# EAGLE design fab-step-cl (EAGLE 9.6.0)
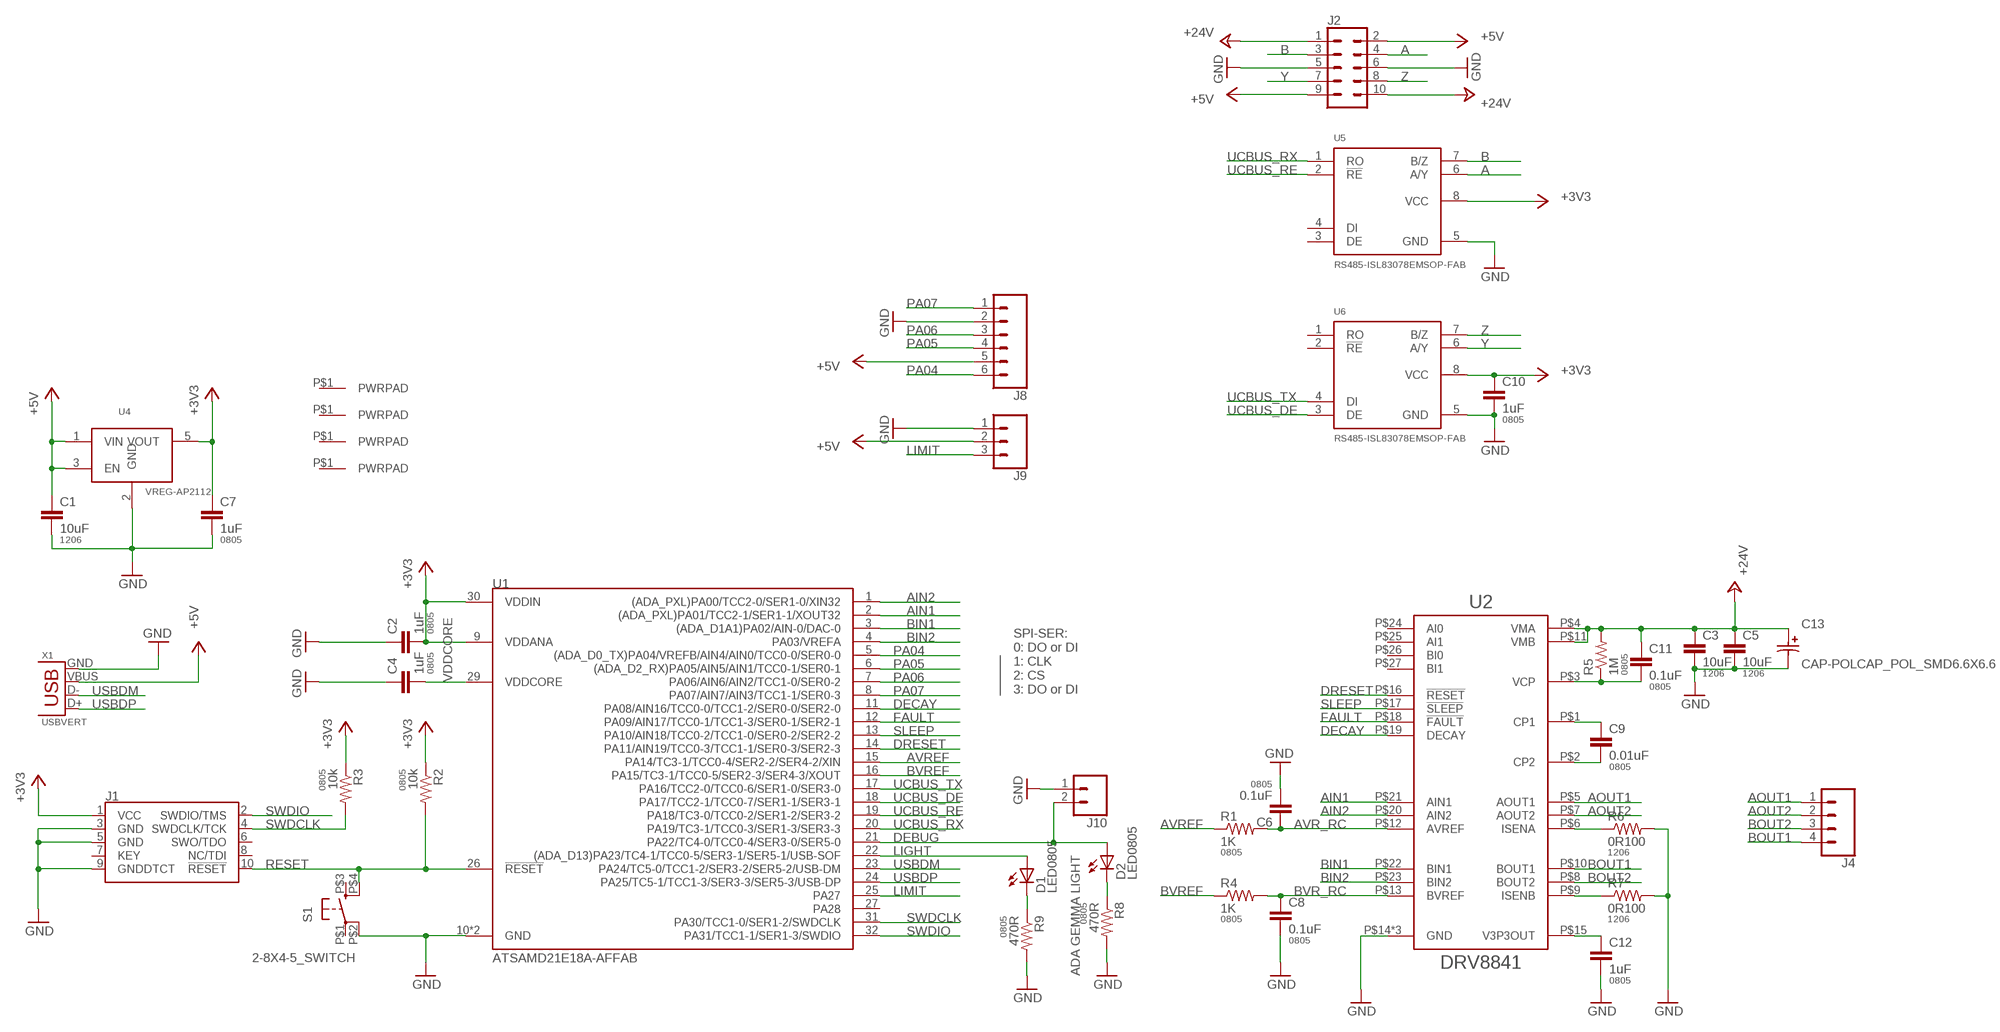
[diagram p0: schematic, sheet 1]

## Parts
C1  10uF  CAP1206  [1206]
C2  1uF  CAP0805  [0805]
C3  10uF  CAP1206  [1206]
C4  1uF  CAP0805  [0805]
C5  10uF  CAP1206  [1206]
C6  0.1uF  CAP0805  [0805]
C7  1uF  CAP0805  [0805]
C8  0.1uF  CAP0805  [0805]
C9  0.01uF  CAP0805  [0805]
C10  1uF  CAP0805  [0805]
C11  0.1uF  CAP0805  [0805]
C12  1uF  CAP0805  [0805]
C13  CAP-POLCAP_POL_SMD6.6X6.6  [SMD-ELEC-CAP]
D1  LED0805  [LED0805]
D2  LED0805  [LED0805]
J1  CORTEX_JTAG_DEBUG_PTH  [2X5-PTH-1.27MM]
J2  CONN_05X2SHD_LOCK_LATCH  [2X5-SHROUDED_LOCK_LATCH]
J3  PWRPADM3  [PWRPAD_3-25MM]
J4  CONN_041X04_NO_SILK  [1X04_NO_SILK]
J5  PWRPADM3  [PWRPAD_3-25MM]
J6  PWRPADM3  [PWRPAD_3-25MM]
J7  PWRPADM3  [PWRPAD_3-25MM]
J8  CONN_06NO_SILK_FEMALE_PTH  [1X06_NO_SILK]
J9  CONN_03JST-PTH-NS  [JST-3-PTH-NS]
J10  CONN_02LOCK  [1X02_LOCK]
R1  1K  RESISTOR0805-RES  [0805]
R2  10k  RESISTOR0805-RES  [0805]
R3  10k  RESISTOR0805-RES  [0805]
R4  1K  RESISTOR0805-RES  [0805]
R5  1M  RESISTOR0805-RES  [0805]
R6  0R100  RESISTOR1206  [1206]
R7  0R100  RESISTOR1206  [1206]
R8  470R  RESISTOR0805-RES  [0805]
R9  470R  RESISTOR0805-RES  [0805]
S1  2-8X4-5_SWITCH  [TACT-SWITCH-KMR6]
U1  ATSAMD21E18A-AFFAB  [TQFP-32-FAB]
U2  DRV8841  [HTSSOP-28]
U4  VREG-AP2112  [SOT23-5]
U5  RS485-ISL83078EMSOP-FAB  [8-MSOP-FAB]
U6  RS485-ISL83078EMSOP-FAB  [8-MSOP-FAB]
X1  USBVERT  [MOLEX_1051330021]

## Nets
+3V3: C2.2 C7.1 C10.1 J1.1(VCC) R2.1 R3.1 U1.9(VDDANA) U1.30(VDDIN) U4.5(VOUT) U5.8(VCC) U6.8(VCC)
+5V: C1.1 J2.2 J2.9 J8.5 J9.2 U4.1(VIN) U4.3(EN) X1.VBUS
+24V: C3.1 C5.1 C11.1 C13.A J2.1 J2.10 R5.2 U2.P$4(VMA) U2.P$11(VMB)
A: J2.4 U5.6(A/Y)
AIN1: U1.2((ADA_PXL)PA01/TCC2-1/SER1-1/XOUT32) U2.P$21(AIN1)
AIN2: U1.1((ADA_PXL)PA00/TCC2-0/SER1-0/XIN32) U2.P$20(AIN2)
AOUT1: J4.1 U2.P$5(AOUT1)
AOUT2: J4.2 U2.P$7(AOUT2)
AVR_RC: C6.1 R1.2 U2.P$12(AVREF)
AVREF: R1.1 U1.15(PA14/TC3-1/TCC0-4/SER2-2/SER4-2/XIN)
B: J2.3 U5.7(B/Z)
BIN1: U1.3((ADA_D1A1)PA02/AIN-0/DAC-0) U2.P$22(BIN1)
BIN2: U1.4(PA03/VREFA) U2.P$23(BIN2)
BOUT1: J4.4 U2.P$10(BOUT1)
BOUT2: J4.3 U2.P$8(BOUT2)
BVR_RC: C8.1 R4.2 U2.P$13(BVREF)
BVREF: R4.1 U1.16(PA15/TC3-1/TCC0-5/SER2-3/SER4-3/XOUT)
DEBUG: D2.1(A) J10.2 U1.21(PA22/TC4-0/TCC0-4/SER3-0/SER5-0)
DECAY: U1.11(PA08/AIN16/TCC0-0/TCC1-2/SER0-0/SER2-0) U2.P$19(DECAY)
DRESET: U1.14(PA11/AIN19/TCC0-3/TCC1-1/SER0-3/SER2-3) U2.P$16(!RESET)
FAULT: U1.12(PA09/AIN17/TCC0-1/TCC1-3/SER0-1/SER2-1) U2.P$18(!FAULT)
GND: C1.2 C2.1 C3.2 C4.1 C5.2 C6.2 C7.2 C8.2 C10.2 C12.2 C13.C J1.3(GND) J1.5(GND) J1.9(GNDDTCT) J2.5 J2.6 J8.2 J9.1 J10.1 R6.2 R7.2 R8.2 R9.2 S1.P$2(P1) U1.10(GND) U1.28(GND) U2.P$14(GND) U2.P$28(GND) U2.P$29(GND) U4.2(GND) U5.5(GND) U6.5(GND) X1.GND
ISENA: R6.1 U2.P$6(ISENA)
ISENB: R7.1 U2.P$9(ISENB)
LIGHT: D1.1(A) U1.22((ADA_D13)PA23/TC4-1/TCC0-5/SER3-1/SER5-1/USB-SOF)
LIMIT: J9.3 U1.25(PA27)
N$1: C9.2 U2.P$2(CP2)
N$2: C9.1 U2.P$1(CP1)
N$3: D2.2(C) R8.1
N$5: C11.2 R5.1 U2.P$3(VCP)
N$6: D1.2(C) R9.1
N$12: C12.1 U2.P$15(V3P3OUT)
PA04: J8.6 U1.5((ADA_D0_TX)PA04/VREFB/AIN4/AIN0/TCC0-0/SER0-0)
PA05: J8.4 U1.6((ADA_D2_RX)PA05/AIN5/AIN1/TCC0-1/SER0-1)
PA06: J8.3 U1.7(PA06/AIN6/AIN2/TCC1-0/SER0-2)
PA07: J8.1 U1.8(PA07/AIN7/AIN3/TCC1-1/SER0-3)
RESET: J1.10(!RESET) R2.2 S1.P$4(S1) U1.26(!RESET)
SLEEP: U1.13(PA10/AIN18/TCC0-2/TCC1-0/SER0-2/SER2-2) U2.P$17(!SLEEP)
SWDCLK: J1.4(SWDCLK/TCK) R3.2 U1.31(PA30/TCC1-0/SER1-2/SWDCLK)
SWDIO: J1.2(SWDIO/TMS) U1.32(PA31/TCC1-1/SER1-3/SWDIO)
UCBUS_DE: U1.18(PA17/TCC2-1/TCC0-7/SER1-1/SER3-1) U6.3(DE)
UCBUS_RE: U1.19(PA18/TC3-0/TCC0-2/SER1-2/SER3-2) U5.2(!RE)
UCBUS_RX: U1.20(PA19/TC3-1/TCC0-3/SER1-3/SER3-3) U5.1(RO)
UCBUS_TX: U1.17(PA16/TCC2-0/TCC0-6/SER1-0/SER3-0) U6.4(DI)
USBDM: U1.23(PA24/TC5-0/TCC1-2/SER3-2/SER5-2/USB-DM) X1.D-
USBDP: U1.24(PA25/TC5-1/TCC1-3/SER3-3/SER5-3/USB-DP) X1.D+
VDDCORE: C4.2 U1.29(VDDCORE)
Y: J2.7 U6.6(A/Y)
Z: J2.8 U6.7(B/Z)
Unconnected: J1.6(SWO/TDO) J1.7(KEY) J1.8(NC/TDI) J3.P$1(PWRPAD) J5.P$1(PWRPAD) J6.P$1(PWRPAD) J7.P$1(PWRPAD) S1.P$1(P) S1.P$3(S) U1.27(PA28) U2.P$24(AI0) U2.P$25(AI1) U2.P$26(BI0) U2.P$27(BI1) U5.3(DE) U5.4(DI) U6.1(RO) U6.2(!RE)

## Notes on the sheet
- SPI-SER:
  0: DO or DI
  1: CLK
  2: CS
  3: DO or DI
- ADA GEMMA LIGHT

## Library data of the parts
C1 C3 C5 = passives:CAP: Capacitor; PACKAGE: 1206
C2 C4 C6-C12 = passives:CAP: Capacitor; PACKAGE: 0805
C13 = passives:CAP-POL
D1 D2 = lights:LED: LED
J1 = SparkFun-Connectors:CORTEX_JTAG_DEBUG: Cortex Debug Connector - 10 pin Supports JTAG debug, Serial Wire debug, and Serial Wire Viewer. PTH and SMD connector options available. General Connector Information Products: PTH Connector -via Digi-Key SparkFun PSoc SparkFun T
J2 = SparkFun-Connectors:CONN_05X2: Multi connection point. Often used as Generic Header-pin footprint for 0.1 inch spaced/style header connections For AVR SPI programming port, see special device with nice symbol: "AVR_SPI_PROG_5x2.dev" You can populate with any combo of single row headers, but if you'd like an exact match, check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
J3 J5-J7 = connector:PWRPAD
J4 = SparkFun-Connectors:CONN_04: Multi connection point. Often used as Generic Header-pin footprint for 0.1 inch spaced/style header connections On any of the 0.1 inch spaced packages, you can populate with these: Break Away Headers - Straight (PRT-00116) Break Away Male Headers - Right Angle (PRT-00553) Female Headers (PRT-00115)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; PROD_ID: CONN-09696
J8 = SparkFun-Connectors:CONN_06: Multi connection point. Often used as Generic Header-pin footprint for 0.1 inch spaced/style header connections On any of the 0.1 inch spaced packages, you can populate with these: Break Away Headers - Straight (PRT-00116) Break Away Male Headers - Right Angle (PRT-00553) Female Headers (PRT-00115)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; PROD_ID: CONN-08437
J9 = SparkFun-Connectors:CONN_03: Multi connection point. Often used as Generic Header-pin footprint for 0.1 inch spaced/style header connections On any of the 0.1 inch spaced packages, you can populate with these: Break Away Headers - Straight (PRT-00116) Break Away Male Headers - Right Angle (PRT-00553) Female Headers (PRT-00115)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
J10 = SparkFun-Connectors:CONN_02: Multi connection point. Often used as Generic Header-pin footprint for 0.1 inch spaced/style header connections
R1-R5 R8 R9 = passives:RESISTOR: Resistor; PACKAGE: 0805
R6 R7 = passives:RESISTOR: Resistor; PACKAGE: 1206
S1 = passives:2-8X4-5_SWITCH
U1 = microcontrollers:ATSAMD21E18A-AF: The SAM D21 is a series of low-power microcontrollers using the 32-bit ARM® Cortex® -M0+ processor, and ranging from 32- to 64-pins with up to 256KB Flash and 32KB of SRAM. The SAM D21 operate at a maximum frequency of 48MHz and reach 2.46 CoreMark® /MHz. Check prices
U2 = power:DRV8841
U4 = power:VREG-AP2112
U5 U6 = comm:RS485-ISL83078E
X1 = connector:USB: SMD micro USB connector as found in the fablab inventory. Three footprint variants included: 609-4613-1-ND used by Jake original, as described by manufacturer's datasheet for milling with the 1/100" bit for milling with the 1/64" bit Made by Zaerc.

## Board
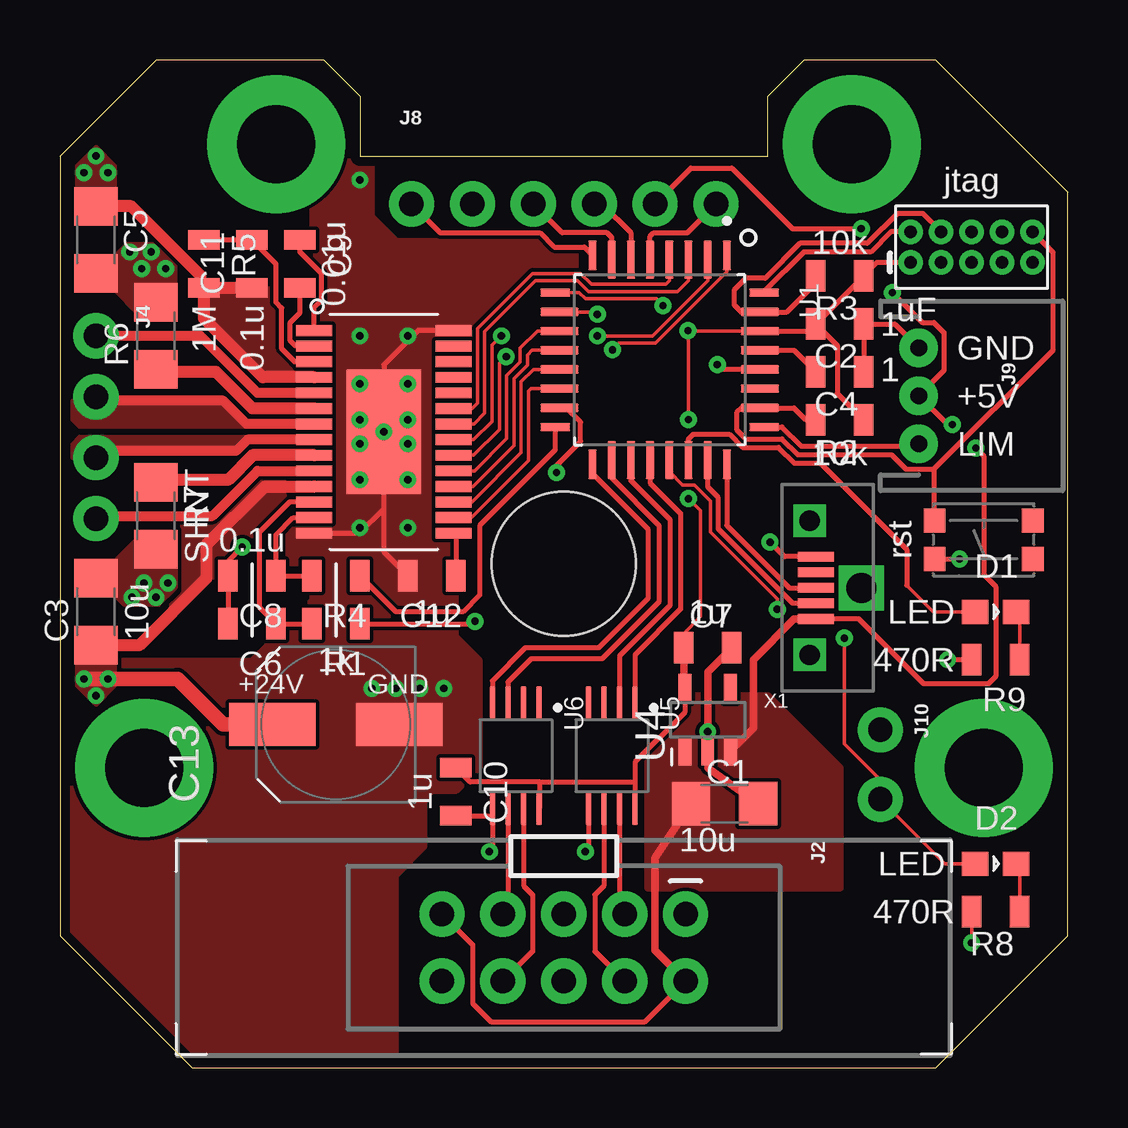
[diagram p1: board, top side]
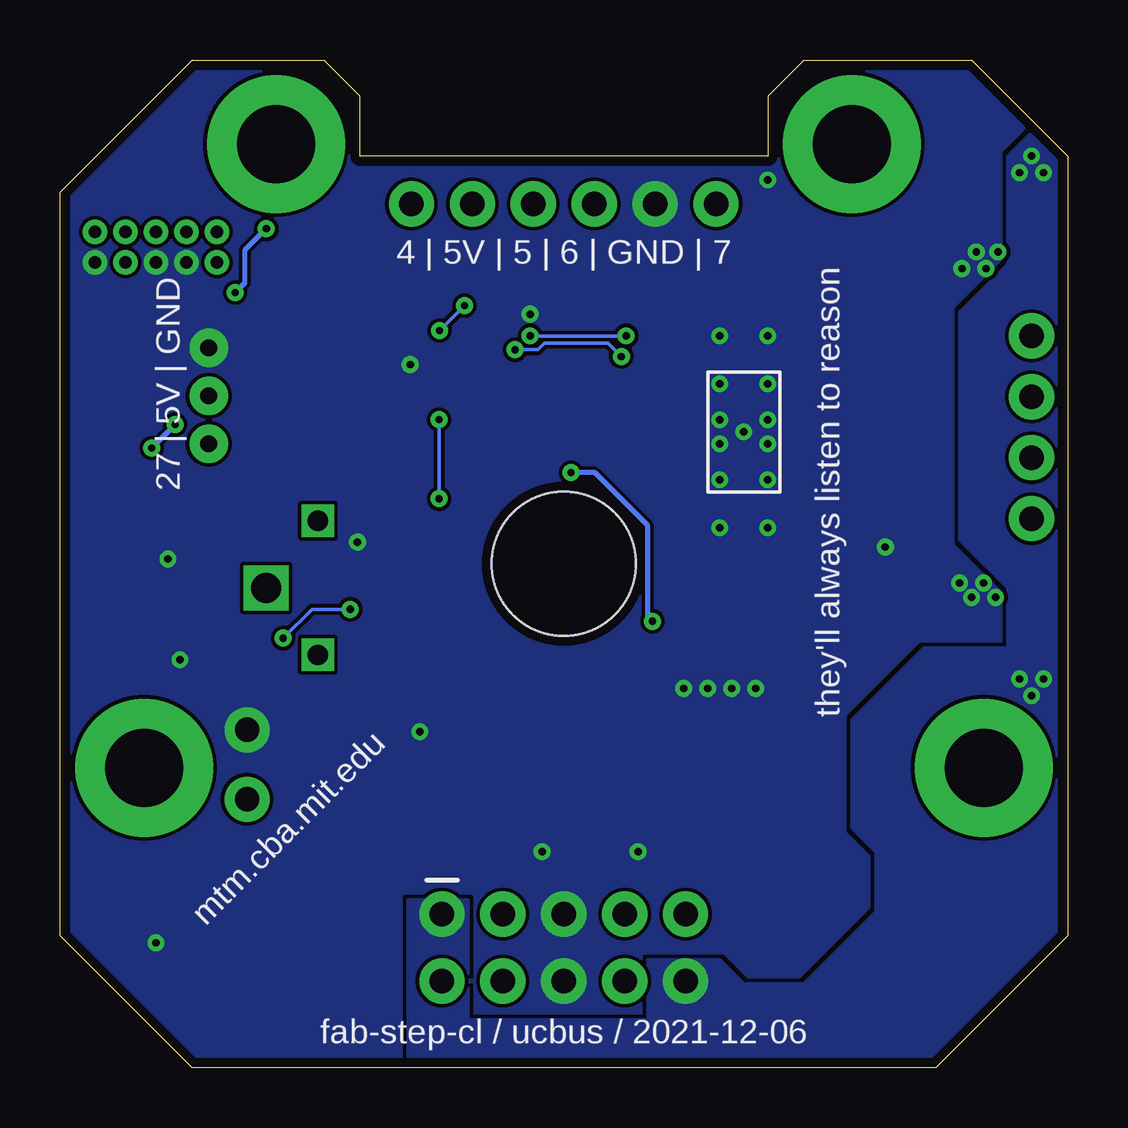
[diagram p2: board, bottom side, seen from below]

Size 42 x 42 mm. Coordinates in mm from the lower left corner, seen from the top.
Outline: 5.5,0 36.5,0 42,5.5 42,36.5 36.5,42 31,42 29.5,40.5 29.5,38 12.5,38 12.5,40.5 11,42 4,42 0,38 0,5.5 5.5,0
Copper layers (1*16): Top 0.035mm / dielectric 1.5mm / Bottom 0.035mm
Design rules "fab *": minimum track width 6mil, minimum drill 0.3mm, track to track 6mil, track to pad 6mil, pad to pad 6mil, via to via 6mil, smd to smd 6mil, copper to edge 16mil, drill to drill 16mil, minimum pad ring 10mil, minimum via ring 8mil, stop-mask expansion 4mil, vias tented up to drill 35mil, thermal gap 16mil
Holes 6 mm at 21,21

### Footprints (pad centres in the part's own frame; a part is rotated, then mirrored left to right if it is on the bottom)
1206 = smd 1.6 x 1.8: 1 -1.4,0; 2 1.4,0
0805 = smd 0.8 x 1.3: 1 -1,0; 2 1,0
SMD-ELEC-CAP = smd 1.8 x 3.6: A 0,2.65; C 0,-2.65
LED0805 = smd 1.1 x 1: 1 -0.85,0; 2 0.85,0
2X5-PTH-1.27MM = drill 0.508 pad 1: 1 -2.54,-0.635; 2 -2.54,0.635; 3 -1.27,-0.635; 4 -1.27,0.635; 5 0,-0.635; 6 0,0.635; 7 1.27,-0.635; 8 1.27,0.635; 9 2.54,-0.635; 10 2.54,0.635
2X5-SHROUDED_LOCK_LATCH = drill 1.016 pad 1.88: 1 -1.397,5.08; 2 1.397,5.08; 3 -1.397,2.54; 4 1.397,2.54; 5 -1.397,0; 6 1.397,0; 7 -1.397,-2.54; 8 1.397,-2.54; 9 -1.397,-5.08; 10 1.397,-5.08
PWRPAD_3-25MM = drill 3.25 pad 5.75: P$1 0,0
1X04_NO_SILK = drill 1.016 pad 1.88: 1 0,0; 2 2.54,0; 3 5.08,0; 4 7.62,0
1X06_NO_SILK = drill 1.016 pad 1.88: 1 0,0; 2 2.54,0; 3 5.08,0; 4 7.62,0; 5 10.16,0; 6 12.7,0
JST-3-PTH-NS = drill 0.7 pad 1.6: 1 -2,0; 2 0,0; 3 2,0
1X02_LOCK = drill 1.016 pad 1.88: 1 -0.178,0; 2 2.718,0
TACT-SWITCH-KMR6 = smd 0.9 x 1: P$1 -2.05,0.8; P$2 2.05,0.8; P$3 -2.05,-0.8; P$4 2.05,-0.8
TQFP-32-FAB = smd 1.25 x 0.35: 1 -4.355,2.8; 8 -4.355,-2.8; 17 4.355,-2.8; 24 4.355,2.8 | smd 1.6 x 0.35: 2 -4.18,2; 3 -4.18,1.2; 4 -4.18,0.4; 5 -4.18,-0.4; 6 -4.18,-1.2; 7 -4.18,-2; 18 4.18,-2; 19 4.18,-1.2; 20 4.18,-0.4; 21 4.18,0.4; 22 4.18,1.2; 23 4.18,2 | smd 0.35 x 1.25: 9 -2.8,-4.355; 16 2.8,-4.355; 25 2.8,4.355; 32 -2.8,4.355 | smd 0.35 x 1.6: 10 -2,-4.18; 11 -1.2,-4.18; 12 -0.4,-4.18; 13 0.4,-4.18; 14 1.2,-4.18; 15 2,-4.18; 26 2,4.18; 27 1.2,4.18; 28 0.4,4.18; 29 -0.4,4.18; 30 -1.2,4.18; 31 -2,4.18
HTSSOP-28 = smd 1.5 x 0.45: P$1 -2.9,4.225; P$2 -2.9,3.575; P$3 -2.9,2.925; P$4 -2.9,2.275; P$5 -2.9,1.625; P$6 -2.9,0.975; P$7 -2.9,0.325; P$8 -2.9,-0.325; P$9 -2.9,-0.975; P$10 -2.9,-1.625; P$11 -2.9,-2.275; P$12 -2.9,-2.925; P$13 -2.9,-3.575; P$14 -2.9,-4.225; P$15 2.9,-4.225; P$16 2.9,-3.575; P$17 2.9,-2.925; P$18 2.9,-2.275; P$19 2.9,-1.625; P$20 2.9,-0.975; P$21 2.9,-0.325; P$22 2.9,0.325; P$23 2.9,0.975; P$24 2.9,1.625; P$25 2.9,2.275; P$26 2.9,2.925; P$27 2.9,3.575; P$28 2.9,4.225 | smd 3.1 x 5.18: P$29 0,0
SOT23-5 = smd 0.533 x 1.194: 1 -0.95,-1.306; 2 0,-1.306; 3 0.95,-1.306; 4 0.95,1.306; 5 -0.95,1.306
8-MSOP-FAB = smd 1.4 x 0.22: 1 -2.2,0.975; 2 -2.2,0.325; 3 -2.2,-0.325; 4 -2.2,-0.975; 5 2.2,-0.975; 6 2.2,-0.325; 7 2.2,0.325; 8 2.2,0.975
MOLEX_1051330021 = smd 0.4 x 1.5: D+ 0,0; D- -0.65,0; GND 1.3,0; ID 0.65,0; VBUS -1.3,0 | drill 0.85 square: P$1 -2.8,0.25; P$2 2.8,0.25 | drill 1.25 square: P$3 0,-1.9

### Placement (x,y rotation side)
C1  27.7,11 0 top
C2  32.5,31 180 top
C3  1.5,19 90 top
C4  32.5,29 180 top
C5  1.5,34.5 270 top
C6  8,18.5 180 top
C7  27,17.5 0 top
C8  8,20.5 180 top
C9  10,33.5 270 top
C10  16.5,11.5 270 top
C11  8,33.5 90 top
C12  15.5,20.5 180 top
C13  11.5,14.3 90 top
D1  39,19 0 top
D2  39,8.5 0 top
J1  38,34.2 0 top
J2  21,5 270 top
J3  9,38.5 0 top
J4  1.5,30.5 270 top
J5  38.5,12.5 0 top
J6  3.5,12.5 0 top
J7  33,38.5 0 top
J8  14.65,36 0 top
J9  35.8,28 270 top
J10  34.2,13.9 270 top
R1  11.5,18.5 180 top
R2  32.5,27 180 top
R3  32.5,33 180 top
R4  11.5,20.5 180 top
R5  6,33.5 270 top
R6  4,30.5 90 top
R7  4,23 270 top
R8  39,6.5 180 top
R9  39,17 180 top
S1  38.5,22 180 top
U1  25,29.5 270 top
U2  13.5,26.5 0 top
U4  27,14.5 0 top
U5  23,13 270 top
U6  19,13 270 top
X1  31.5,20 90 top

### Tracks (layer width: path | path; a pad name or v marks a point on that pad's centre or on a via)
+3V3  (via drill 0.3)
  Top 0.152: U1.9 21.64,32.3 21.9,32.04 24.86,32.04 v25.14,31.76 | U1.30 26.2,30.7 | 26.2,30.7 v26.18,30.72 | C7.1 26,18.1 26.7,18.8 26.7,23.21 v26.2,23.71 | v26.2,27.01 26.2,30.7
  Top 0.203: U1.30 31.2,30.7 C2.2 | C2.2 R3.1 34.06,33.56 J1.1 | C2.2 32.4,30.1 32.4,28.1 R2.1 | U6.8 20,10.82 20,11.9 | U4.5 26.05,14.81 23.98,12.73 23.98,11.9 | 23.98,11.9 U5.8 | 20,11.9 23.98,11.9 | 20,11.9 17.1,11.9 C10.1
  Top 0.305: U4.5 26,15.86 C7.1
  Bottom 0.152: v25.14,31.76 v26.18,30.72 | v26.2,23.71 v26.2,27.01
+5V  (via drill 0.3)
  Top 0.203: v34.7,32.3 35.95,31.05 36.44,31.05 36.85,30.64 36.85,29.05 J9.2 37,26.8 v37.2,26.8 | J8.5 26.3,37.49 28.01,37.49 30.54,34.96 v33.4,34.96 | J2.9 17.2,5.12 17.2,2.67 17.97,1.91 24.39,1.91 J2.2 | v38.17,25.82 38.5,25.5 38.5,20.56 39,20.06 39,16.3 38.7,16 36,16 33.3,18.7 X1.VBUS
  Top 0.305: J2.2 24.8,4.88 24.8,8.75 C1.1 | X1.VBUS 30.6,18.7 28.9,17 28.9,14.14 U4.3
  Bottom 0.203: v33.4,34.96 34.3,34.06 34.3,32.7 v34.7,32.3 | v37.2,26.8 v38.17,25.82
  pour Top (rank 2, no thermals): 24.5,15.5 24.5,7.5 32.5,7.5 32.5,12.5 29.5,15.5
+24V  (via drill 0.3)
  Top 0.508: U2.P$11 10.58,24.21 8.53,24.21 6.1,21.77 6.1,20.4 3.3,17.6 C3.1 | U2.P$4 8.45,28.77 6,31.22 R5.2 | C11.1 R5.2 | R5.2 5.86,32.64 5.86,33.02 2.97,35.9 C5.1
  Top 0.61: C13.A 6.8,14.3 4.9,16.2 v1,16.2
  other vias: 2,37.3 1,37.3 1.5,38 2,16.2 1.5,15.5
  pour Top (rank 2, no thermals): 0.7,35.2 0.7,37.6 1.5,38.4 2.3,37.6 2.3,35.2
  pour Top (no thermals): 2.3,18.3 2.3,15.9 1.5,15.1 0.7,15.9 0.7,18.3
  pour Bottom: -1.5,14.5 1.5,14.5 2.5,15.5 2.5,20 4.5,22 4.5,31.5 2.5,33.5 2.5,38 1,39.5 -1,39.5 -1,16 -1.5,15.5
  pour Bottom (no thermals): 25,7 25,2 17.5,2 17.5,4.5 14.5,4.5 13.5,3.5 11,3.5 8,6.5 8,9 9,10 9,14.5 6,17.5 -1,17.5 -2.5,16 -2.5,-1.5 -2,-2 27.5,-2 27.5,7
  pour Top (no thermals): 10.3,28.8 10.3,32.5 6.4,32.5 6,32.1 6,31.2 8.4,28.8
  pour Top (rank 3): 10.3,24.2 9.1,23 9.1,22.7 6.8,20.4 6.3,20.4 5.2,19.3 4,19.3 4,22 4.9,22.9 6.4,22.9 8.3,24.8 10.3,24.8
A
  Top 0.203: U5.6 22.68,7.58 22.3,7.2 22.3,4.84 J2.4
AIN1  (via drill 0.3)
  Top 0.152: U1.2 27,32.8 24.7,30.5 v22.4,30.5 | U2.P$21 17.25,26.18 18.01,26.94 18.01,30.11 v18.4,30.5
  Bottom 0.152: v22.4,30.5 v18.4,30.5
AIN2  (via drill 0.3)
  Top 0.152: U1.1 27.8,33.17 24.83,30.2 23.31,30.2 v23.03,29.92 | v18.6,29.64 18.31,29.36 18.31,26.59 17.25,25.52 U2.P$20
  Bottom 0.152: v23.03,29.92 22.08,29.92 21.8,30.2 19.15,30.2 v18.6,29.64
AOUT1
  Top 0.406: U2.P$5 8.24,28.12 5.86,30.5 J4.1
AOUT2
  Top 0.406: U2.P$7 7.78,26.82 6.8,27.8 1.66,27.8 J4.2
  pour Top (rank 3, no thermals): 8,26.7 0.8,26.7 0.5,27 0.5,27.8 6.8,27.8 7.7,26.9 8,26.9
AVR_RC
  Top 0.203: U2.P$12 9.57,23.57 8.3,22.3 8.3,19.2 C6.1 R1.2
AVREF  (via drill 0.3)
  Top 0.203: R1.1 17.2,18.5 v17.3,18.6 | v20.7,24.8 20.7,25.1 21.7,26.1 21.7,26.9 21.1,27.5 U1.15
  Bottom 0.203: v17.3,18.6 17.49,18.79 17.49,22.59 19.7,24.8 v20.7,24.8
B
  Top 0.203: U5.7 23.32,6.61 J2.3
BIN1
  Top 0.152: U2.P$22 17.26,26.82 17.7,27.27 17.7,30.67 19.83,32.8 21.57,32.8 22.02,32.35 25.75,32.35 26.2,32.8 U1.3
BIN2
  Top 0.152: U1.4 25.4,32.8 25.25,32.65 22.15,32.65 21.7,33.1 19.7,33.1 17.4,30.8 17.4,27.7 17.18,27.48 U2.P$23
BOUT1
  Top 0.406: U2.P$10 8.24,24.88 6.36,23 1.62,23 J4.4
BOUT2
  Top 0.406: U2.P$8 7.81,26.18 7.34,25.7 1.78,25.7 J4.3
  pour Top (rank 3, no thermals): 7.9,26.3 0.8,26.3 0.5,26 0.5,25.4 1.6,25.4 1.8,25.6 7.2,25.6
BVR_RC
  Top 0.203: R4.2 C8.1 9,22.2 9.72,22.93 U2.P$13
BVREF
  Top 0.203: U1.16 20.64,25.75 17.49,22.59 17.49,19.69 16.8,19 14,19 R4.1
DEBUG  (via drill 0.3)
  Top 0.152: U1.21 25.4,24.85 25.96,24.29 26.44,24.29 27.11,23.62 27.11,22.32 29.9,19.53 v29.9,19.1 | v32.7,17.9 32.7,13.48 34.2,11.98 J10.2 36.88,8.5 D2.1
  Bottom 0.152: v29.9,19.1 31.5,19.1 v32.7,17.9
DECAY
  Top 0.152: U1.11 19.9,30.7 19.18,29.98 19.18,29.4 18.62,28.84 18.62,26.22 17.27,24.88 U2.P$19
DRESET
  Top 0.152: U1.14 19.63,28.3 19.53,28.2 19.53,25.3 17.16,22.93 U2.P$16
FAULT
  Top 0.152: U1.12 19.69,29.9 19.49,29.7 19.49,29.27 18.92,28.71 18.92,25.92 17.23,24.23 U2.P$18
GND  (via drill 0.3)
  Top 0.152: U1.10 22.3,31.5 v22.4,31.4 | R8.2 v38,5.2
  Top 0.203: U1.28 27.6,29.1 v27.4,29.3 | C4.1 C2.1 34.8,31 J9.1 | U6.5 18.02,10.5 | 18.02,10.5 18.02,9.12 v17.9,9 | U5.5 22.02,9.12 v21.9,9 | S1.P$2 v37.5,21.2 | R9.2 v37,17 | X1.GND 30.2,21.3 v29.6,21.9 | C10.2 18.02,10.5 | U2.P$14 12.47,22.27 13.5,23.3 | 13.5,23.3 U2.P$29 13.5,29.3 14.93,30.73 U2.P$28 | C12.2 13.5,21.5 13.5,23.3 | C6.2 C8.2 7,21.1 v7.6,21.7
  Top 0.305: C1.2 27,12.5 U4.2 v27,14 27,16.5 C7.2
  other vias: 4.4,33.3 3.8,34 3.4,33.3 3.5,20.2 4,19.6 4.5,20.2 16,15.8 15,15.8 14,15.8 13,15.8 12.5,26 12.5,27 12.5,28.5 14.5,28.5 14.5,27 14.5,26 14.5,24.5 12.5,24.5 13.5,26.5 12.5,30.5 14.5,30.5 14.5,22.5 12.5,22.5 12.5,37 2.9,34 3,19.6
  pour Bottom (rank 2, no thermals): -0.5,43 42.5,43 42.5,-0.5 -0.5,-0.5
  pour Top (rank 2, no thermals): 13,44 13,35.5 14,34.5 20,34.5 20.5,34 21.5,34 21.5,33 20,33 16.5,29.5 16.5,18 17.5,17 17.5,12.5 16.5,11.5 15.5,11.5 15.2,11.2 15.2,9.2 14,8 14,-1 3.5,-1 -1,3.5 -1,17 8,17 10.5,19.5 10.5,21 9.5,21 9.5,23 10.5,24 10.5,44
  pour Top (rank 2, no thermals): 0.7,21.1 2.3,21.1 3.5,22.3 4.8,22.3 4.8,20 4.1,19.3 2.7,19.3 2.3,19.7 0.7,19.7
  pour Top (rank 2, no thermals): 4.8,31.2 4.8,33.5 4,34.3 2.8,34.3 2.3,33.8 0.7,33.8 0.7,32.4 2.3,32.4 3.2,31.5 3.2,31.2
ISENA
  Top 0.508: R6.1 4,29 6.5,29 8.03,27.48 U2.P$6
ISENB
  Top 0.508: R7.1 4,24.5 7,24.5 8.03,25.52 U2.P$9
LIGHT
  Top 0.152: 35.3,20.1 36.4,19 D1.1
  Top 0.203: U1.22 26.2,26.2 26.4,26.4 27.9,26.4 28.45,25.84 29.95,25.84 30.61,25.19 31.7,25.19 35.3,21.59 35.3,20.1
LIMIT
  Top 0.203: U1.25 30.1,26.7 30.9,25.9 35.7,25.9 J9.3
N$1
  Top 0.203: U2.P$2 9.82,30.07 9.6,30.3 9.6,31.05 10,31.46 C9.2
N$2
  Top 0.203: U2.P$1 10.6,31.69 10.9,32 10.9,33.1 10,34 C9.1
N$3
  Top 0.152: D2.2 40,8.35 R8.1
N$5
  Top 0.203: U2.P$3 9.78,29.43 9.24,29.96 9.24,31.66 9,31.9 9,33.5 C11.2 R5.1
N$6
  Top 0.152: D1.2 40,18.85 R9.1
N$12
  Top 0.203: U2.P$15 16.5,22.18 C12.1
PA04
  Top 0.203: U1.5 24.6,34.65 24.75,34.8 26.15,34.8 J8.6
PA05
  Top 0.203: J8.4 22.6,36 23.8,34.8 U1.6
PA06
  Top 0.203: U1.7 23,34.6 22.8,34.8 20.93,34.8 J8.3
PA07
  Top 0.203: J8.1 15.85,34.8 20,34.8 20.6,34.2 21.86,34.2 U1.8
RESET
  Top 0.203: R2.2 31.1,27 30.6,27.5 U1.26 28.4,27.5 28.2,27.3 28.2,26.6 28.6,26.2 30.1,26.2 30.75,25.54 34.66,25.54 35.26,24.95 36.44,24.95 | 36.44,24.95 41.4,29.91 41.4,33.98 J1.10 | 36.44,24.95 36.44,22.81 S1.P$4
SLEEP
  Top 0.152: U1.13 19.74,29.1 19.23,28.59 19.23,25.63 17.18,23.57 U2.P$17
SWDCLK
  Top 0.203: R3.2 31.5,32.7 30.3,31.5 U1.31 28.4,31.5 28.1,31.8 28.1,32.4 28.6,32.9 29.4,32.9 30.85,34.36 33.65,34.36 34.9,35.6 35.97,35.6 J1.4
SWDIO
  Top 0.203: J1.2 34.63,34.84 33.8,34 31,34 29.36,32.35 U1.32
UCBUS_DE
  Top 0.203: U1.18 23,24.56 24.96,22.6 24.96,19.4 22.6,17.04 19.64,17.04 18.68,16.07 U6.3
UCBUS_RE
  Top 0.203: U1.19 23.8,24.47 25.42,22.85 25.42,19.25 23.32,17.16 U5.2
UCBUS_RX
  Top 0.203: U1.20 24.6,24.37 25.88,23.09 25.88,19.11 23.98,17.2 U5.1
UCBUS_TX
  Top 0.203: U1.17 22.2,24.76 24.51,22.45 24.51,19.55 22.45,17.49 19.39,17.49 18.02,16.12 U6.4
USBDM
  Top 0.203: X1.D- 30.55,19.35 27.44,22.45 27.44,23.76 27,24.2 U1.23
USBDP
  Top 0.203: X1.D+ 30.4,20 27.8,22.6 U1.24
VDDCORE
  Top 0.203: U1.29 30.6,29.9 C4.2
Y
  Top 0.203: U6.6 18.68,6.61 J2.7
Z
  Top 0.203: U6.7 19.32,7.58 19.7,7.2 19.7,4.84 J2.8

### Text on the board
tPlace: jtag | 0.01u | 10k | 1M | 0.1u | uF | 1 | GND | 1 | +5V | 10k | LIM | SHNT | 0.1u | rst | 10u | 1u | 1u | LED | 1k | 470R | +24V | GND | 1u | 10u | LED | 470R
bPlace: 4 | 5V | 5 | 6 | GND | 7 | 27 | 5V | GND | they'll always listen to reason | mtm.cba.mit.edu | fab-step-cl / ucbus / 2021-12-06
